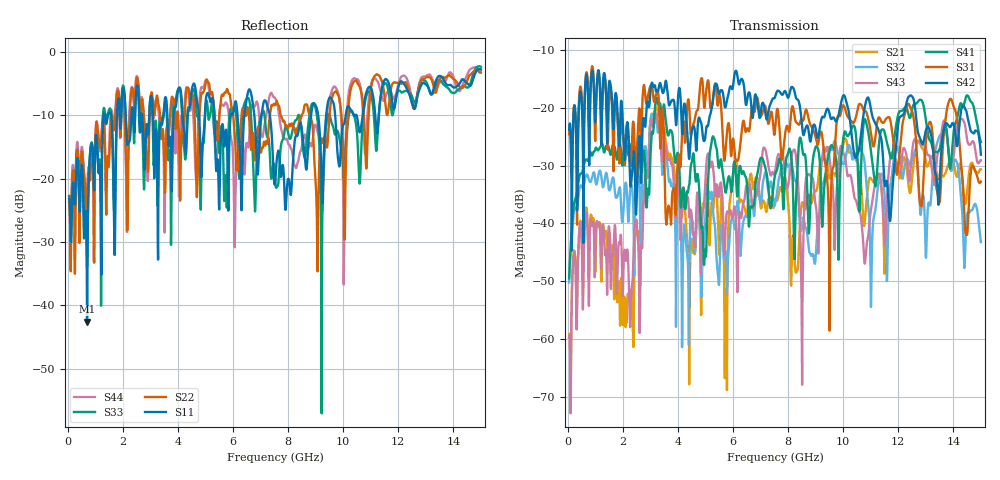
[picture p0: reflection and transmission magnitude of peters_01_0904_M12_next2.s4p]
# MHZ S RI R 50.00
! FREQ  S11  S12  S13  S14
!  S21  S22  S23  S24
!  S31  S32  S33  S34
!  S41  S42  S43  S44
!  REAL  IMAG  REAL  IMAG  REAL  IMAG  REAL  IMAG
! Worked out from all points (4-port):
!   1496 points, 50 MHz to 15 GHz, reference 50 ohm
!   strongest paths, dB at 50 MHz, 3.79 GHz, 7.53 GHz, 11.27 GHz, 15 GHz:
!     S42: -23.8, -18.7, -18.1, -23.7, -28.1
!     S31: -24.6, -35.1, -23.6, -21.8, -32.8
!     S41: -49.5, -24.4, -31.6, -28.1, -25.9
!     S43: -59.7, -29.9, -31.0, -31.4, -29.1
!     S32: -50.2, -33.1, -36.6, -33.4, -43.3
!     S21: -59.9, -28.7, -35.9, -31.6, -30.7
!   lowest |S11| = -42.6 dB at 700 MHz (marker M1), VSWR 1.01, Z = 49.3 - j0.239 ohm
!   |S11| at or under -10 dB: start of sweep to 1.301 GHz; 5.321 GHz to 5.918 GHz (597 MHz wide, 10.6 % of centre); 7.34 GHz to 8.834 GHz (1.494 GHz wide, 18.5 % of centre)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
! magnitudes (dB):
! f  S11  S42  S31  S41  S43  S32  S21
! 50 MHz  -23.2  -23.8  -24.6  -49.5  -59.7  -50.2  -59.9
! 700 MHz  -42.6  -14.6  -14.1  -29.1  -39.1  -31.5  -38.1
! 2.33 GHz  -9.1  -31.7  -26.3  -26.2  -50.8  -33.7  -52.4
! 3.62 GHz  -10.3  -17.2  -38.5  -24.4  -28.9  -29.9  -27.5
! 5.74 GHz  -12.3  -19.7  -26.8  -34.7  -39.8  -45.7  -52.7
! 6.08 GHz  -7.8  -13.7  -28.6  -30.0  -37.6  -41.1  -29.3
! 15 GHz  -2.7  -28.1  -32.8  -25.9  -29.1  -43.3  -30.7
